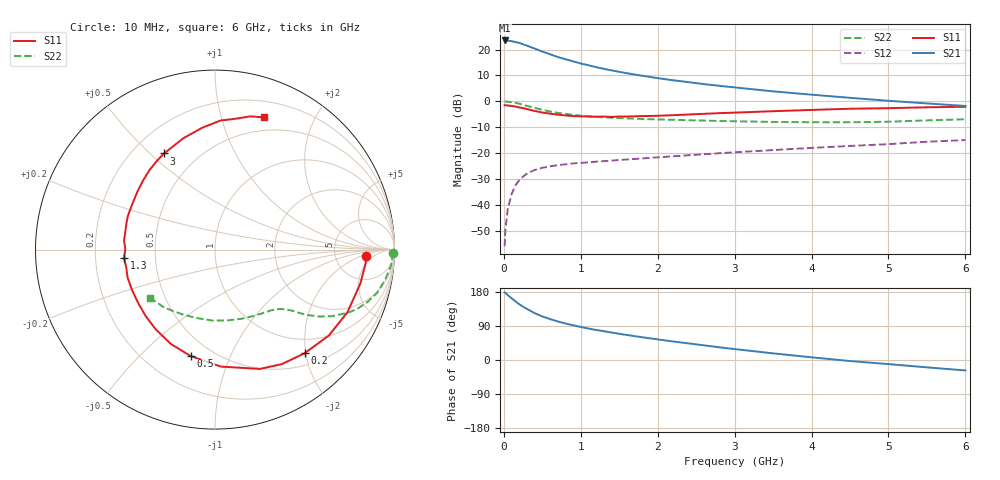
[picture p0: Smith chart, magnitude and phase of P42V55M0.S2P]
! SIEMENS Small Signal Semiconductors
! BFP182
! Si NPN RF Bipolar Junction Transistor in SOT143
! VCE = 2.5 V  IC = 5 mA
! Common Emitter S-Parameters:  March  1996
# GHz  S  MA  R  50
!  f  S11  S21  S12  S22
! GHz  MAG  ANG  MAG  ANG  MAG  ANG  MAG  ANG
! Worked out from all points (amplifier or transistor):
!   36 points, 10 MHz to 6 GHz, reference 50 ohm
!   highest |S21| = 23.5 dB at 10 MHz (marker M1)
!   |S21| within 3 dB of that: start of sweep to 389.2 MHz
!   unconditionally stable (mu >= 1): 1.579 GHz to 5.468 GHz
!   at 250 MHz: K = 0.21, MSG = 25.5 dB, |S12| = -29.1 dB
!   at 1.4 GHz: K = 0.94, MSG = 17.4 dB, |S12| = -22.9 dB
!   at 6 GHz: K = 0.95, MSG = 6.6 dB, |S12| = -15.0 dB
!   lowest NFmin = 1.20 dB at 450 MHz
!   S11 on the Smith chart (normalised r, x): 10 MHz: 11, -3; 200 MHz: 0.71, -1.97; 500 MHz: 0.38, -0.72; 1.3 GHz: 0.33, -0.04; 3 GHz: 0.33, +0.55; 6 GHz: 0.36, +1.38
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0.01  0.8403 -2.4  14.98 178.4  0.0016 89.5  0.9901 -1.0
0.02  0.843 -5.0  14.94 177.1  0.0033 82.5  0.9892 -2.0
0.05  0.8319 -13.0  14.94 171.4  0.0082 86.1  0.9846 -5.2
0.1  0.8164 -25.3  14.51 163.0  0.0161 75.2  0.9621 -10.2
0.15  0.7946 -37.1  13.97 155.0  0.0238 70.3  0.9357 -14.8
0.2  0.7632 -49.2  13.45 147.3  0.03 65.4  0.8993 -18.9
0.25  0.7388 -59.7  12.61 140.6  0.0352 60.4  0.8586 -22.6
0.3  0.7102 -69.4  11.88 134.9  0.0402 55.9  0.8206 -25.4
0.4  0.6527 -87.1  10.46 123.7  0.0473 49.4  0.7478 -29.8
0.5  0.6086 -102.8  9.144 114.9  0.0521 44.3  0.686 -32.9
0.6  0.5803 -115.1  8.135 108.0  0.0556 40.8  0.6374 -35.0
0.7  0.5531 -126.9  7.181 101.9  0.0587 38.6  0.6011 -36.4
0.8  0.5343 -136.6  6.507 96.4  0.0608 36.6  0.572 -37.5
1.1  0.5114 -162.2  4.971 83.0  0.0665 34.1  0.5134 -40.4
1.3  0.5085 -174.6  4.244 75.9  0.0701 33.2  0.4908 -42.3
1.7  0.5139 164.0  3.292 63.0  0.0773 32.7  0.4621 -47.0
2.2  0.5398 143.2  2.552 48.9  0.0869 32.6  0.4407 -54.2
3  0.606 117.9  1.86 28.8  0.1038 30.7  0.4131 -68.9
3.5  0.6453 105.8  1.56 17.5  0.1147 28.9  0.4007 -79.8
4.5  0.72 87.5  1.17 -2.7  0.1378 24.4  0.3946 -104.8
5.5  0.768 75.2  0.912 -19.4  0.1663 19.0  0.4289 -130.9
6  0.7859 69.5  0.815 -27.6  0.1786 14.7  0.4514 -143.5
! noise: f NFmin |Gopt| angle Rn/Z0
0.45  1.2  0.27  37  0.3
0.9  1.3  0.25  75  0.23
1.8  1.9  0.21  145  0.2
